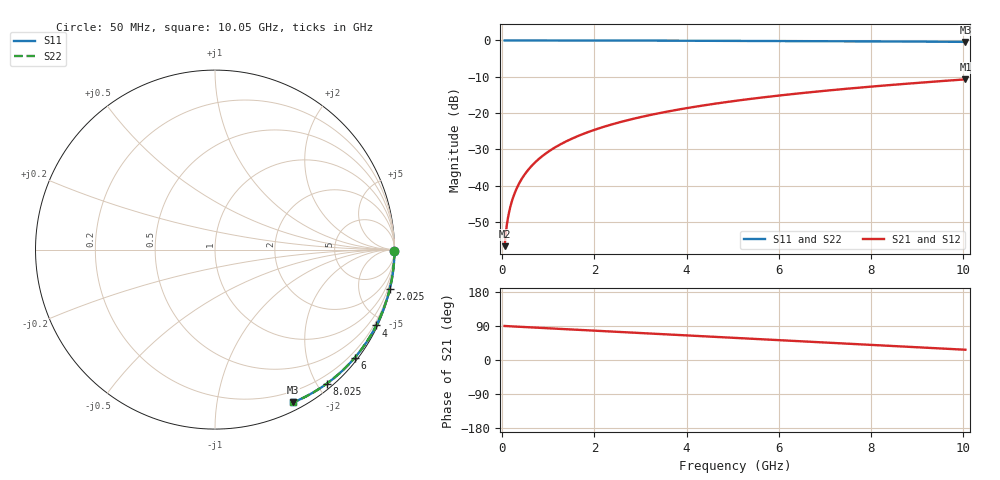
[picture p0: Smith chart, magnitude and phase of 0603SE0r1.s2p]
! AVX Thin Film Operation		Date: August 2001
! Description: Accu-P® Series, Thin Film, SMD, RF Capacitor
! Part Number: 06035J0R1ABT
! 50 MHz  -  10.05 GHz
! Serial Measurements
# mhz S db R 50
!	S11		S21		S12		S22
!	dB	Phase	dB	Phase	dB	Phase	dB	Phase
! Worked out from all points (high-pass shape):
!   401 points, 50 MHz to 10.05 GHz, reference 50 ohm
!   highest |S21| = -10.71 dB at 10.05 GHz (marker M1); lowest = -56.6 dB at 50 MHz (marker M2)
!   |S21| within 3 dB of the highest: 7.123 GHz to end of sweep
!   lowest |S11| = -0.4 dB at 10.05 GHz (marker M3), VSWR 44.55, Z = 4.12 - j81.7 ohm
!   |S11| at or under -10 dB: nowhere
!   |S22| runs from -0.4 to 0.0 dB; largest |S21 - S12| = 0
!   S11 on the Smith chart (normalised r, x): 50 MHz: open; 2.025 GHz: 0.07, -8.93; 4 GHz: 0.07, -4.48; 6 GHz: 0.07, -2.93; 8.025 GHz: 0.08, -2.13; 10.05 GHz: 0.08, -1.63
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50  -0.00 -0.3  -56.62 89.8  -56.62 89.8  -0.00 -0.3
75  -0.00 -0.5  -53.10 89.7  -53.10 89.7  -0.00 -0.5
125  -0.00 -0.8  -48.67 89.3  -48.67 89.3  -0.00 -0.8
150  -0.00 -0.9  -47.08 89.1  -47.08 89.1  -0.00 -0.9
225  -0.00 -1.4  -43.56 88.6  -43.56 88.6  -0.00 -1.4
275  -0.00 -1.7  -41.82 88.3  -41.82 88.3  -0.00 -1.7
350  -0.00 -2.2  -39.72 87.8  -39.72 87.8  -0.00 -2.2
500  -0.00 -3.2  -36.62 86.9  -36.62 86.9  -0.00 -3.2
725  -0.00 -4.6  -33.40 85.4  -33.40 85.4  -0.00 -4.6
1000  -0.00 -6.3  -30.61 83.7  -30.61 83.7  -0.00 -6.3
1325  -0.01 -8.4  -28.17 81.6  -28.17 81.6  -0.01 -8.4
1725  -0.01 -10.9  -25.88 79.1  -25.88 79.1  -0.01 -10.9
2025  -0.02 -12.8  -24.49 77.2  -24.49 77.2  -0.02 -12.8
2650  -0.03 -16.7  -22.17 73.3  -22.17 73.3  -0.03 -16.7
3400  -0.04 -21.4  -20.02 68.6  -20.02 68.6  -0.04 -21.4
4000  -0.06 -25.2  -18.63 64.8  -18.63 64.8  -0.06 -25.2
5050  -0.10 -31.7  -16.64 58.2  -16.64 58.2  -0.10 -31.7
6000  -0.14 -37.7  -15.17 52.3  -15.17 52.3  -0.14 -37.6
6725  -0.17 -42.2  -14.20 47.8  -14.20 47.8  -0.17 -42.1
8025  -0.24 -50.2  -12.68 39.7  -12.68 39.7  -0.24 -50.2
8400  -0.27 -52.5  -12.29 37.4  -12.29 37.4  -0.27 -52.5
10050  -0.39 -62.8  -10.71 27.1  -10.71 27.1  -0.39 -62.8
